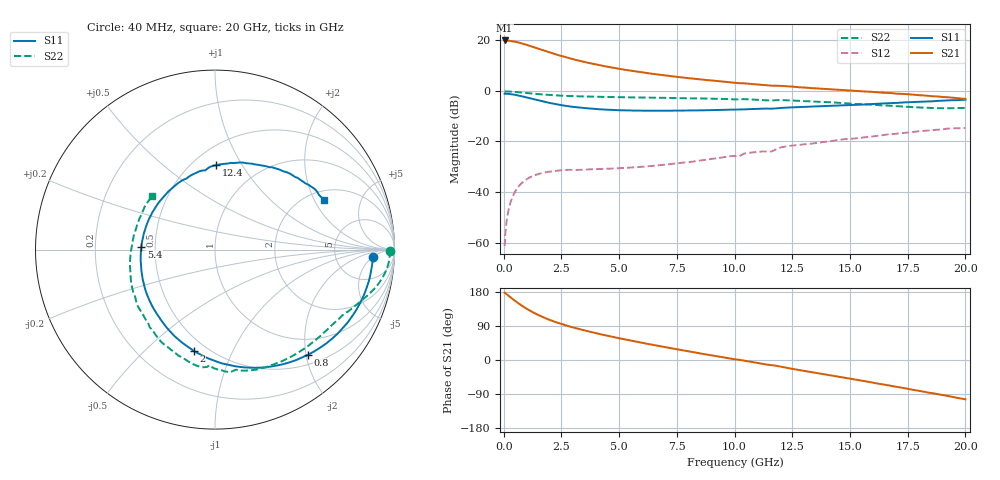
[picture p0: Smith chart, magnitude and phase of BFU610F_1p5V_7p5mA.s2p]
! Filename:  P:\Prog\Test\Noise\ATS_data\Testdata_Net\SplitFiles\BFU610_2W_A5_HighFreq_1.5V_7.5mA_D.s2p
! Date/Time: Wed 10/Aug/2011 16:54:20
! BFU610_2W_A5_HighFreq_Bias5_1.5V_1mA_10mA_R.s2p
! MDIF S-parameter v. bias file
! BFU610_2W_A5_HighFreq_1.5V_1mA_10mA
! Date/time Mon Aug 08 13:57:57 2011
! VAR V_out= 1.5002
! VAR I_out= 7.4950
! VAR V_in= 0.9248
! VAR I_in= 0.0673
! Device data file deembeded for feedlines and parallel
! Original file: \SplitFiles\BFU610_2W_A5_HighFreq_1.5V_7.5mA_R.s2p
! Feed-files: PR003V01_101208_Feed1.s2p, PR003V01_101208_Feed2.s2p
! Parallel-file: PR003V01_101208_Par.s2p
# MHz S MA R 50
!  Freq-MHz  S11-mag  S11-arg  S21-mag  S21-arg  S12-mag  S12-arg  S22-mag  S22-arg
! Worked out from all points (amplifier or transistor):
!   167 points, 40 MHz to 20 GHz, reference 50 ohm
!   highest |S21| = 20.0 dB at 40 MHz (marker M1)
!   |S21| within 3 dB of that: start of sweep to 1.415 GHz
!   unconditionally stable (mu >= 1): 48.58 MHz to 50.58 MHz; 2.473 GHz to end of sweep
!   at 550 MHz: K = 0.23, MSG = 29.2 dB, |S12| = -39.0 dB
!   at 4.2 GHz: K = 1.77, MAG = 15.4 dB, |S12| = -30.9 dB
!   at 20 GHz: K = 1.65, MAG = 1.0 dB, |S12| = -14.7 dB
!   S11 on the Smith chart (normalised r, x): 40 MHz: 14, -5; 800 MHz: 0.67, -2.03; 2 GHz: 0.43, -0.72; 5.4 GHz: 0.42, +0.02; 12.4 GHz: 0.64, +0.78; 20 GHz: 2.43, +2.41
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40  0.8806 -2.6  9.962 178.0  0.0008472 81.8  0.9732 -0.3
100  0.8788 -6.4  9.895 175.0  0.002086 83.5  0.9748 -1.5
180  0.875 -11.6  9.857 171.2  0.003776 83.4  0.9735 -2.9
420  0.8478 -26.6  9.534 159.4  0.008737 75.5  0.9609 -6.9
600  0.8191 -37.4  9.166 151.2  0.01209 69.1  0.9461 -9.5
800  0.7821 -48.6  8.669 142.8  0.01532 62.7  0.9273 -12.2
1050  0.7331 -61.6  7.999 133.3  0.01855 55.8  0.9031 -15.0
1300  0.6859 -73.7  7.342 124.8  0.02111 50.2  0.8803 -17.5
1650  0.6269 -88.5  6.497 114.5  0.0236 43.8  0.853 -20.4
2000  0.5772 -101.6  5.762 105.6  0.02532 39.0  0.832 -23.1
2250  0.548 -110.0  5.3 100.0  0.02597 36.6  0.8172 -25.0
2600  0.5137 -120.9  4.754 93.1  0.02708 33.6  0.8 -27.1
3400  0.4627 -141.9  3.827 79.6  0.0276 30.5  0.7778 -32.3
4300  0.429 -161.8  3.131 66.6  0.02864 30.4  0.7615 -38.2
5400  0.4108 177.7  2.56 52.5  0.03026 33.1  0.7471 -45.7
6800  0.4049 155.4  2.074 36.1  0.03403 37.7  0.7307 -55.6
8800  0.4156 128.3  1.64 14.3  0.04364 42.2  0.7077 -70.6
10200  0.4266 111.7  1.422 0.5  0.05077 44.4  0.6805 -80.6
12400  0.4706 89.3  1.222 -22.3  0.08181 37.9  0.6486 -101.1
13400  0.491 79.7  1.132 -32.5  0.09134 31.9  0.616 -111.3
16800  0.5745 50.4  0.9065 -68.5  0.1393 9.4  0.5066 -156.2
20000  0.6684 24.2  0.695 -103.7  0.1848 -22.4  0.4613 139.6
